| IBIS file stm32h523_533_lqfp144.ibs
[IBIS ver] 4.2
[File name] stm32h523_533_lqfp144.ibs
[File Rev] 0.2
[Date] 07-05-2024
[Source] Data Created at STMicroelectronics
[Notes]  File originated from ELDO simulations.
[Disclaimer]  This information is for modeling purpose only and is
   not guaranteed. The information is subject to change without
   notice.
[Copyright] Copyright 2024 STMicroelectronics Inc.
|   Component stm32h523_533_lqfp144
[Component] stm32h523_533_lqfp144
[Manufacturer] STMicroelectronics
[Package]
| variable   typ   min   max
R_pkg  0  NA  NA
L_pkg  0  NA  NA
C_pkg  0  NA  NA
[Pin]   signal_name   model_name
1  PE2  io8_ft_i3c_spi
2  PE3  io8_ft_i3c_spi
3  PE4  io8_ft_i3c_spi
4  PE5  io8_ft_i3c_spi
5  PE6  io8_ft_i3c_spi
6  VBAT  power
7  PC13  io8_ft_i3c_spi_v33
8  PC14-OSC32_IN  io_ft_tamp
9  PC15-OSC32_OUT  io_ft_tamp
10  PF0  io8_ft_i3c_spi
11  PF1  io8_ft_i3c_spi
12  PF2  io8_ft_i3c_spi
13  PF3  io8_ft_i3c_spi
14  PF4  io8_ft_i3c_spi
15  PF5  io8_ft_i3c_spi
16  VSS  gnd
17  VDD  power
18  PF6  io8_ft_i3c_spi
19  PF7  io8_ft_i3c_spi
20  PF8  io8_ft_i3c_spi
21  PF9  io8_ft_i3c_spi
22  PF10  io8_ft_i3c_spi
23  PH0-OSC_IN  io8_ft_i3c_spi
24  PH1-OSC_OUT  io8_ft_i3c_spi
25  NRST  ioreset_ft_v33
26  PC0  io8_ft_spi
27  PC1  io8_ft_spi
28  PC2  io8_ft_spi
29  PC3  io8_ft_spi
30  VDD  power
31  VSSA  nc
32  VREFP  nc
33  VDDA  nc
34  PA0  io8_ft_spi
35  PA1  io8_ft_spi_tamp
36  PA2  io8_ft_spi
37  PA3  io8_ft_spi
38  VSS  gnd
39  VDD  power
40  PA4  io8_ft_spi
41  PA5  io8_ft_spi
42  PA6  io8_ft_spi
43  PA7  io8_ft_spi
44  PC4  io8_ft_spi
45  PC5  io8_ft_spi
46  PB0  io8_ft_spi
47  PB1  io8_ft_spi
48  PB2  io8_ft_i3c_spi
49  PF11  io8_ft_spi
50  PF12  io8_ft_spi
51  VSS  gnd
52  VDD  power
53  PF13  io8_ft_spi
54  PF14  io8_ft_spi
55  PF15  io8_ft_i3c_spi
56  PG0  io8_ft_i3c_spi
57  PG1  io8_ft_i3c_spi
58  PE7  io8_ft_i3c_spi
59  PE8  io8_ft_i3c_spi
60  PE9  io8_ft_i3c_spi
61  VSS  gnd
62  VDD  power
63  PE10  io8_ft_i3c_spi
64  PE11  io8_ft_i3c_spi
65  PE12  io8_ft_i3c_spi
66  PE13  io8_ft_i3c_spi
67  PE14  io8_ft_i3c_spi
68  PE15  io8_ft_i3c_spi
69  PB10  io8_ft_i3c_spi
70  VCAP  nc
71  VSS  gnd
72  VDD  power
73  PB12  io8_ft_i3c_spi
74  PB13  nc
75  PB14  nc
76  PB15  io8_ft_spi
77  PD8  io8_ft_i3c_spi
78  PD9  io8_ft_i3c_spi
79  PD10  io8_ft_i3c_spi
80  PD11  io8_ft_i3c_spi
81  PD12  io8_ft_i3c_spi
82  PD13  io8_ft_i3c_spi
83  VSS  gnd
84  VDD  power
85  PD14  io8_ft_i3c_spi
86  PD15  io8_ft_i3c_spi
87  PG2  io8_ft_i3c_spi
88  PG3  io8_ft_i3c_spi
89  PG4  io8_ft_i3c_spi
90  PG5  io8_ft_i3c_spi
91  PG6  io8_ft_i3c_spi
92  PG7  io8_ft_i3c_spi
93  PG8  io8_ft_i3c_spi
94  VSS  gnd
95  VDD  power
96  PC6  io8_ft_i3c_spi
97  PC7  io8_ft_i3c_spi
98  PC8  io8_ft_i3c_spi
99  PC9  io8_ft_i3c_spi
100  PA8  io8_ft_i3c_spi
101  PA9  io8_ft_i3c_spi
102  PA10  io8_ft_i3c_spi
103  PA11  io8usb_ft_i3c_spi_phy
104  PA12  io8usb_ft_i3c_spi_phy
105  PA13  io8_ft_i3c_spi
106  VDDUSB  power
107  VSS  gnd
108  VDD  power
109  PA14  io8_ft_i3c_spi
110  PA15  io8_ft_i3c_spi
111  PC10  io8_ft_i3c_spi
112  PC11  io8_ft_i3c_spi
113  PC12  io8_ft_i3c_spi
114  PD0  io8_ft_i3c_spi
115  PD1  io8_ft_i3c_spi
116  PD2  io8_ft_i3c_spi
117  PD3  io8_ft_i3c_spi
118  PD4  io8_ft_i3c_spi
119  PD5  io8_ft_i3c_spi
120  VSS  gnd
121  VDDIO2  power
122  PD6  io8_ft_i3c_spi
123  PD7  io8_ft_i3c_spi
124  PG9  io8_ft_i3c_spi
125  PG10  io8_ft_i3c_spi
126  PG11  io8_ft_i3c_spi
127  PG12  io8_ft_i3c_spi
128  PG13  io8_ft_i3c_spi
129  PG14  io8_ft_i3c_spi
130  VSS  gnd
131  VDD  power
132  PG15  io8_ft_i3c_spi
133  PB3  io8_ft_i3c_spi
134  PB4  io8_ft_i3c_spi
135  PB5  io8_ft_i3c_spi
136  PB6  io8_ft_i3c_spi
137  PB7  io8_ft_i3c_spi
138  BOOT0  vpphv
139  PB8  io8_ft_i3c_spi
140  PB9  io8_ft_i3c_spi
141  PE0  io8_ft_i3c_spi
142  VCAP  nc
143  VSS  gnd
144  VDD  power
[Package Model]   478-lqfp-20x20-144-240315
[Pin Mapping]   pulldown_ref   pullup_ref   | Comment
1  gndio  vddio
2  gndio  vddio
3  gndio  vddio
4  gndio  vddio
5  gndio  vddio
6  nc  vsw
7  gndio  vddio  | Depending on IO usage
| 7  gndio  vsw  | Depending on IO usage
8  gndio  vddio  | Depending on IO usage
| 8  gndio  vsw  | Depending on IO usage
9  gndio  vddio  | Depending on IO usage
| 9  gndio  vsw  | Depending on IO usage
10  gndio  vddio
11  gndio  vddio
12  gndio  vddio
13  gndio  vddio
14  gndio  vddio
15  gndio  vddio
16  gndio  nc
17  nc  vddio
18  gndio  vddio
19  gndio  vddio
20  gndio  vddio
21  gndio  vddio
22  gndio  vddio
23  gndio  vddio
24  gndio  vddio
25  gndio  vddio
26  gndio  vddio
27  gndio  vddio
28  gndio  vddio
29  gndio  vddio
30  nc  vddio
31  nc  nc
32  nc  nc
33  nc  nc
34  gndio  vddio
35  gndio  vddio
36  gndio  vddio
37  gndio  vddio
38  gndio  nc
39  nc  vddio
40  gndio  vddio
41  gndio  vddio
42  gndio  vddio
43  gndio  vddio
44  gndio  vddio
45  gndio  vddio
46  gndio  vddio
47  gndio  vddio
48  gndio  vddio
49  gndio  vddio
50  gndio  vddio
51  gndio  nc
52  nc  vddio
53  gndio  vddio
54  gndio  vddio
55  gndio  vddio
56  gndio  vddio
57  gndio  vddio
58  gndio  vddio
59  gndio  vddio
60  gndio  vddio
61  gndio  nc
62  nc  vddio
63  gndio  vddio
64  gndio  vddio
65  gndio  vddio
66  gndio  vddio
67  gndio  vddio
68  gndio  vddio
69  gndio  vddio
70  nc  nc
71  gndio  nc
72  nc  vddio
73  gndio  vddio
74  nc  nc
75  nc  nc
76  gndio  vddio
77  gndio  vddio
78  gndio  vddio
79  gndio  vddio
80  gndio  vddio
81  gndio  vddio
82  gndio  vddio
83  gndio  nc
84  nc  vddio
85  gndio  vddio
86  gndio  vddio
87  gndio  vddio
88  gndio  vddio
89  gndio  vddio
90  gndio  vddio
91  gndio  vddio
92  gndio  vddio
93  gndio  vddio
94  gndio  nc
95  nc  vddio
96  gndio  vddio
97  gndio  vddio
98  gndio  vddio
99  gndio  vddio
100  gndio  vddio
101  gndio  vddio
102  gndio  vddio
103  gndio  vddusb  | Depending on IO usage
| 103  gndio  vddio  | Depending on IO usage
104  gndio  vddusb  | Depending on IO usage
| 104  gndio  vddio  | Depending on IO usage
105  gndio  vddio
106  nc  vddusb
107  gndio  nc
108  nc  vddio
109  gndio  vddio
110  gndio  vddio
111  gndio  vddio
112  gndio  vddio
113  gndio  vddio
114  gndio  vddio
115  gndio  vddio
116  gndio  vddio
117  gndio  vddio
118  gndio  vddio
119  gndio  vddio
120  gndio  nc
121  nc  vddmmc
122  gndio  vddmmc
123  gndio  vddmmc
124  gndio  vddmmc
125  gndio  vddmmc
126  gndio  vddmmc
127  gndio  vddmmc
128  gndio  vddmmc
129  gndio  vddmmc
130  gndio  nc
131  nc  vddio
132  gndio  vddio
133  gndio  vddio
134  gndio  vddio
135  gndio  vddio
136  gndio  vddio
137  gndio  vddio
138  gndio  vddio
139  gndio  vddmmc
140  gndio  vddmmc
141  gndio  vddio
142  nc  nc
143  gndio  nc
144  nc  vddio
|[Diff Pin]  inv_pin  vdiff  tdelay_typ  tdelay_min  tdelay_max
|104  103  NA  NA  NA  NA
[Model Selector] io8_ft_i3c_spi
io8_ft_spi_ls_1v2 "GPIO SPI - 5V tolerant - low speed - 1.2V range"
io8_ft_spi_ls_1v8 "GPIO SPI - 5V tolerant - low speed - 1.8V range"
io8_ft_spi_ls_3v3 "GPIO SPI - 5V tolerant - low speed - 3.3V range"
io8_ft_spi_ms_1v2 "GPIO SPI - 5V tolerant - med speed - 1.2V range"
io8_ft_spi_ms_1v8 "GPIO SPI - 5V tolerant - med speed - 1.8V range"
io8_ft_spi_ms_3v3 "GPIO SPI - 5V tolerant - med speed - 3.3V range"
io8_ft_spi_fs_1v2 "GPIO SPI - 5V tolerant - fast speed - 1.2V range"
io8_ft_spi_fs_1v8 "GPIO SPI - 5V tolerant - fast speed - 1.8V range"
io8_ft_spi_fs_3v3 "GPIO SPI - 5V tolerant - fast speed - 3.3V range"
io8_ft_spi_hs_1v2 "GPIO SPI - 5V tolerant - high speed - 1.2V range"
io8_ft_spi_hs_1v8 "GPIO SPI - 5V tolerant - high speed - 1.8V range"
io8_ft_spi_hs_3v3 "GPIO SPI - 5V tolerant - high speed - 3.3V range"
io8_ft_hslv_spi_ls_1v2 "GPIO SPI low volt opt - 5V tolerant - low speed - 1.2V range"
io8_ft_hslv_spi_ls_1v8 "GPIO SPI low volt opt - 5V tolerant - low speed - 1.8V range"
io8_ft_hslv_spi_ls_2v5 "GPIO SPI low volt opt - 5V tolerant - low speed - 2.5V range"
io8_ft_hslv_spi_ms_1v2 "GPIO SPI low volt opt - 5V tolerant - med speed - 1.2V range"
io8_ft_hslv_spi_ms_1v8 "GPIO SPI low volt opt - 5V tolerant - med speed - 1.8V range"
io8_ft_hslv_spi_ms_2v5 "GPIO SPI low volt opt - 5V tolerant - med speed - 2.5V range"
io8_ft_hslv_spi_fs_1v2 "GPIO SPI low volt opt - 5V tolerant - fast speed - 1.2V range"
io8_ft_hslv_spi_fs_1v8 "GPIO SPI low volt opt - 5V tolerant - fast speed - 1.8V range"
io8_ft_hslv_spi_fs_2v5 "GPIO SPI low volt opt - 5V tolerant - fast speed - 2.5V range"
io8_ft_hslv_spi_hs_1v2 "GPIO SPI low volt opt - 5V tolerant - high speed - 1.2V range"
io8_ft_hslv_spi_hs_1v8 "GPIO SPI low volt opt - 5V tolerant - high speed - 1.8V range"
io8_ft_hslv_spi_hs_2v5 "GPIO SPI low volt opt - 5V tolerant - high speed - 2.5V range"
io8_ft_i3c_spi_ls_1v2 "GPIO SPI with I3C open-drain - 5V tolerant - low speed - 1.2V range"
io8_ft_i3c_spi_ls_1v8 "GPIO SPI with I3C open-drain - 5V tolerant - low speed - 1.8V range"
io8_ft_i3c_spi_ls_3v3 "GPIO SPI with I3C open-drain - 5V tolerant - low speed - 3.3V range"
io8_ft_i3c_spi_ms_1v2 "GPIO SPI with I3C open-drain - 5V tolerant - med speed - 1.2V range"
io8_ft_i3c_spi_ms_1v8 "GPIO SPI with I3C open-drain - 5V tolerant - med speed - 1.8V range"
io8_ft_i3c_spi_ms_3v3 "GPIO SPI with I3C open-drain - 5V tolerant - med speed - 3.3V range"
io8_ft_i3c_spi_fs_1v2 "GPIO SPI with I3C open-drain - 5V tolerant - fast speed - 1.2V range"
io8_ft_i3c_spi_fs_1v8 "GPIO SPI with I3C open-drain - 5V tolerant - fast speed - 1.8V range"
io8_ft_i3c_spi_fs_3v3 "GPIO SPI with I3C open-drain - 5V tolerant - fast speed - 3.3V range"
io8_ft_i3c_spi_hs_1v2 "GPIO SPI with I3C open-drain - 5V tolerant - high speed - 1.2V range"
io8_ft_i3c_spi_hs_1v8 "GPIO SPI with I3C open-drain - 5V tolerant - high speed - 1.8V range"
io8_ft_i3c_spi_hs_3v3 "GPIO SPI with I3C open-drain - 5V tolerant - high speed - 3.3V range"
io8_ft_hslv_i3c_spi_ls_1v2 "GPIO SPI low volt opt with I3C open-drain - 5V tolerant - low speed - 1.2V range"
io8_ft_hslv_i3c_spi_ls_1v8 "GPIO SPI low volt opt with I3C open-drain - 5V tolerant - low speed - 1.8V range"
io8_ft_hslv_i3c_spi_ls_2v5 "GPIO SPI low volt opt with I3C open-drain - 5V tolerant - low speed - 2.5V range"
io8_ft_hslv_i3c_spi_ms_1v2 "GPIO SPI low volt opt with I3C open-drain - 5V tolerant - med speed - 1.2V range"
io8_ft_hslv_i3c_spi_ms_1v8 "GPIO SPI low volt opt with I3C open-drain - 5V tolerant - med speed - 1.8V range"
io8_ft_hslv_i3c_spi_ms_2v5 "GPIO SPI low volt opt with I3C open-drain - 5V tolerant - med speed - 2.5V range"
io8_ft_hslv_i3c_spi_fs_1v2 "GPIO SPI low volt opt with I3C open-drain - 5V tolerant - fast speed - 1.2V range"
io8_ft_hslv_i3c_spi_fs_1v8 "GPIO SPI low volt opt with I3C open-drain - 5V tolerant - fast speed - 1.8V range"
io8_ft_hslv_i3c_spi_fs_2v5 "GPIO SPI low volt opt with I3C open-drain - 5V tolerant - fast speed - 2.5V range"
io8_ft_hslv_i3c_spi_hs_1v2 "GPIO SPI low volt opt with I3C open-drain - 5V tolerant - high speed - 1.2V range"
io8_ft_hslv_i3c_spi_hs_1v8 "GPIO SPI low volt opt with I3C open-drain - 5V tolerant - high speed - 1.8V range"
io8_ft_hslv_i3c_spi_hs_2v5 "GPIO SPI low volt opt with I3C open-drain - 5V tolerant - high speed - 2.5V range"
io8_ft_i3c_fmp_spi_3v3 "GPIO SPI with I3C fm+ open-drain - 5V tolerant - 3.3V range"
io8_ft_i3c_fmp_spi_1v8 "GPIO SPI with I3C fm+ open-drain - 5V tolerant - 1.8V range"
io8_ft_i3c_fmp_spi_1v2 "GPIO SPI with I3C fm+ open-drain - 5V tolerant - 1.2V range"
[Model Selector] io8_ft_i3c_spi_v33
io8_ft_spi_v33_ls_1v2 ""GPIO SPI V33 - 5V tolerant - low speed - 1.2V range"
io8_ft_spi_v33_ls_1v8 ""GPIO SPI V33 - 5V tolerant - low speed - 1.8V range"
io8_ft_spi_v33_ls_3v3 ""GPIO SPI V33 - 5V tolerant - low speed - 3.3V range"
io8_ft_spi_v33_ms_1v2 ""GPIO SPI V33 - 5V tolerant - med speed - 1.2V range"
io8_ft_spi_v33_ms_1v8 ""GPIO SPI V33 - 5V tolerant - med speed - 1.8V range"
io8_ft_spi_v33_ms_3v3 ""GPIO SPI V33 - 5V tolerant - med speed - 3.3V range"
io8_ft_spi_v33_fs_1v2 ""GPIO SPI V33 - 5V tolerant - fast speed - 1.2V range
io8_ft_spi_v33_fs_1v8 ""GPIO SPI V33 - 5V tolerant - fast speed - 1.8V range
io8_ft_spi_v33_fs_3v3 ""GPIO SPI V33 - 5V tolerant - fast speed - 3.3V range
io8_ft_spi_v33_hs_1v2 ""GPIO SPI V33 - 5V tolerant - high speed - 1.2V range
io8_ft_spi_v33_hs_1v8 ""GPIO SPI V33 - 5V tolerant - high speed - 1.8V range
io8_ft_spi_v33_hs_3v3 ""GPIO SPI V33 - 5V tolerant - high speed - 3.3V range
io8_ft_hslv_spi_v33_ls_1v2 "GPIO SPI V33 low volt opt - 5V tolerant - low speed - 1.2V range""
io8_ft_hslv_spi_v33_ls_1v8 "GPIO SPI V33 low volt opt - 5V tolerant - low speed - 1.8V range""
io8_ft_hslv_spi_v33_ls_2v5 "GPIO SPI V33 low volt opt - 5V tolerant - low speed - 2.5V range""
io8_ft_hslv_spi_v33_ms_1v2 "GPIO SPI V33 low volt opt - 5V tolerant - med speed - 1.2V range""
io8_ft_hslv_spi_v33_ms_1v8 "GPIO SPI V33 low volt opt - 5V tolerant - med speed - 1.8V range""
io8_ft_hslv_spi_v33_ms_2v5 "GPIO SPI V33 low volt opt - 5V tolerant - med speed - 2.5V range""
io8_ft_hslv_spi_v33_fs_1v2 "GPIO SPI V33 low volt opt - 5V tolerant - fast speed - 1.2V range"
io8_ft_hslv_spi_v33_fs_1v8 "GPIO SPI V33 low volt opt - 5V tolerant - fast speed - 1.8V range"
io8_ft_hslv_spi_v33_fs_2v5 "GPIO SPI V33 low volt opt - 5V tolerant - fast speed - 2.5V range"
io8_ft_hslv_spi_v33_hs_1v2 "GPIO SPI V33 low volt opt - 5V tolerant - high speed - 1.2V range"
io8_ft_hslv_spi_v33_hs_1v8 "GPIO SPI V33 low volt opt - 5V tolerant - high speed - 1.8V range"
io8_ft_hslv_spi_v33_hs_2v5 "GPIO SPI V33 low volt opt - 5V tolerant - high speed - 2.5V range"
io8_ft_i3c_spi_v33_ls_1v2 "GPIO SPI V33 with I3C open-drain - 5V tolerant - low speed - 1.2V range"
io8_ft_i3c_spi_v33_ls_1v8 "GPIO SPI V33 with I3C open-drain - 5V tolerant - low speed - 1.8V range"
io8_ft_i3c_spi_v33_ls_3v3 "GPIO SPI V33 with I3C open-drain - 5V tolerant - low speed - 3.3V range"
io8_ft_i3c_spi_v33_ms_1v2 "GPIO SPI V33 with I3C open-drain - 5V tolerant - med speed - 1.2V range"
io8_ft_i3c_spi_v33_ms_1v8 "GPIO SPI V33 with I3C open-drain - 5V tolerant - med speed - 1.8V range"
io8_ft_i3c_spi_v33_ms_3v3 "GPIO SPI V33 with I3C open-drain - 5V tolerant - med speed - 3.3V range"
io8_ft_i3c_spi_v33_fs_1v2 "GPIO SPI V33 with I3C open-drain - 5V tolerant - fast speed - 1.2V range"
io8_ft_i3c_spi_v33_fs_1v8 "GPIO SPI V33 with I3C open-drain - 5V tolerant - fast speed - 1.8V range"
io8_ft_i3c_spi_v33_fs_3v3 "GPIO SPI V33 with I3C open-drain - 5V tolerant - fast speed - 3.3V range"
io8_ft_i3c_spi_v33_hs_1v2 "GPIO SPI V33 with I3C open-drain - 5V tolerant - high speed - 1.2V range"
io8_ft_i3c_spi_v33_hs_1v8 "GPIO SPI V33 with I3C open-drain - 5V tolerant - high speed - 1.8V range"
io8_ft_i3c_spi_v33_hs_3v3 "GPIO SPI V33 with I3C open-drain - 5V tolerant - high speed - 3.3V range"
io8_ft_hslv_i3c_spi_v33_ls_1v2 "GPIO SPI V33 low volt opt with I3C open-drain - 5V tolerant - low speed - 1.2V range"
io8_ft_hslv_i3c_spi_v33_ls_1v8 "GPIO SPI V33 low volt opt with I3C open-drain - 5V tolerant - low speed - 1.8V range"
io8_ft_hslv_i3c_spi_v33_ls_2v5 "GPIO SPI V33 low volt opt with I3C open-drain - 5V tolerant - low speed - 2.5V range"
io8_ft_hslv_i3c_spi_v33_ms_1v2 "GPIO SPI V33 low volt opt with I3C open-drain - 5V tolerant - med speed - 1.2V range"
io8_ft_hslv_i3c_spi_v33_ms_1v8 "GPIO SPI V33 low volt opt with I3C open-drain - 5V tolerant - med speed - 1.8V range"
io8_ft_hslv_i3c_spi_v33_ms_2v5 "GPIO SPI V33 low volt opt with I3C open-drain - 5V tolerant - med speed - 2.5V range"
io8_ft_hslv_i3c_spi_v33_fs_1v2 "GPIO SPI V33 low volt opt with I3C open-drain - 5V tolerant - fast speed - 1.2V range"
io8_ft_hslv_i3c_spi_v33_fs_1v8 "GPIO SPI V33 low volt opt with I3C open-drain - 5V tolerant - fast speed - 1.8V range"
io8_ft_hslv_i3c_spi_v33_fs_2v5 "GPIO SPI V33 low volt opt with I3C open-drain - 5V tolerant - fast speed - 2.5V range"
io8_ft_hslv_i3c_spi_v33_hs_1v2 "GPIO SPI V33 low volt opt with I3C open-drain - 5V tolerant - high speed - 1.2V range"
io8_ft_hslv_i3c_spi_v33_hs_1v8 "GPIO SPI V33 low volt opt with I3C open-drain - 5V tolerant - high speed - 1.8V range"
io8_ft_hslv_i3c_spi_v33_hs_2v5 "GPIO SPI V33 low volt opt with I3C open-drain - 5V tolerant - high speed - 2.5V range"
io8_ft_i3c_fmp_spi_v33_3v3 "GPIO SPI V33 with I3C fm+ open-drain - 5V tolerant - 3.3V range"
io8_ft_i3c_fmp_spi_v33_1v8 "GPIO SPI V33 with I3C fm+ open-drain - 5V tolerant - 1.8V range"
io8_ft_i3c_fmp_spi_v33_1v2 "GPIO SPI V33 with I3C fm+ open-drain - 5V tolerant - 1.2V range"
[Model Selector] io8_ft_spi
io8_ft_spi_ls_1v2 "GPIO SPI - 5V tolerant - low speed - 1.2V range"
io8_ft_spi_ls_1v8 "GPIO SPI - 5V tolerant - low speed - 1.8V range"
io8_ft_spi_ls_3v3 "GPIO SPI - 5V tolerant - low speed - 3.3V range"
io8_ft_spi_ms_1v2 "GPIO SPI- 5V tolerant - med speed - 1.2V range"
io8_ft_spi_ms_1v8 "GPIO SPI- 5V tolerant - med speed - 1.8V range"
io8_ft_spi_ms_3v3 "GPIO SPI- 5V tolerant - med speed - 3.3V range"
io8_ft_spi_fs_1v2 "GPIO SPI- 5V tolerant - fast speed - 1.2V range"
io8_ft_spi_fs_1v8 "GPIO SPI- 5V tolerant - fast speed - 1.8V range"
io8_ft_spi_fs_3v3 "GPIO SPI- 5V tolerant - fast speed - 3.3V range"
io8_ft_spi_hs_1v2 "GPIO SPI- 5V tolerant - high speed - 1.2V range"
io8_ft_spi_hs_1v8 "GPIO SPI- 5V tolerant - high speed - 1.8V range"
io8_ft_spi_hs_3v3 "GPIO SPI- 5V tolerant - high speed - 3.3V range"
io8_ft_hslv_spi_ls_1v2 "GPIO SPI low volt opt - 5V tolerant - low speed - 1.2V range"
io8_ft_hslv_spi_ls_1v8 "GPIO SPI low volt opt - 5V tolerant - low speed - 1.8V range"
io8_ft_hslv_spi_ls_2v5 "GPIO SPI low volt opt - 5V tolerant - low speed - 2.5V range"
io8_ft_hslv_spi_ms_1v2 "GPIO SPI low volt opt - 5V tolerant - med speed - 1.2V range"
io8_ft_hslv_spi_ms_1v8 "GPIO SPI low volt opt - 5V tolerant - med speed - 1.8V range"
io8_ft_hslv_spi_ms_2v5 "GPIO SPI low volt opt - 5V tolerant - med speed - 2.5V range"
io8_ft_hslv_spi_fs_1v2 "GPIO SPI low volt opt - 5V tolerant - fast speed - 1.2V range"
io8_ft_hslv_spi_fs_1v8 "GPIO SPI low volt opt - 5V tolerant - fast speed - 1.8V range"
io8_ft_hslv_spi_fs_2v5 "GPIO SPI low volt opt - 5V tolerant - fast speed - 2.5V range"
io8_ft_hslv_spi_hs_1v2 "GPIO SPI low volt opt - 5V tolerant - high speed - 1.2V range"
io8_ft_hslv_spi_hs_1v8 "GPIO SPI low volt opt - 5V tolerant - high speed - 1.8V range"
io8_ft_hslv_spi_hs_2v5 "GPIO SPI low volt opt - 5V tolerant - high speed - 2.5V range"
[Model Selector] io8_ft_spi_tamp
io8_ft_spi_ls_1v2 "GPIO SPI - 5V tolerant - low speed - 1.2V range"
io8_ft_spi_ls_1v8 "GPIO SPI - 5V tolerant - low speed - 1.8V range"
io8_ft_spi_ls_3v3 "GPIO SPI- 5V tolerant - low speed - 3.3V range"
io8_ft_spi_ms_1v2 "GPIO SPI - 5V tolerant - med speed - 1.2V range"
io8_ft_spi_ms_1v8 "GPIO SPI - 5V tolerant - med speed - 1.8V range"
io8_ft_spi_ms_3v3 "GPIO SPI - 5V tolerant - med speed - 3.3V range"
io8_ft_spi_fs_1v2 "GPIO SPI - 5V tolerant - fast speed - 1.2V range"
io8_ft_spi_fs_1v8 "GPIO SPI - 5V tolerant - fast speed - 1.8V range"
io8_ft_spi_fs_3v3 "GPIO SPI - 5V tolerant - fast speed - 3.3V range"
io8_ft_spi_hs_1v2 "GPIO SPI - 5V tolerant - high speed - 1.2V range"
io8_ft_spi_hs_1v8 "GPIO SPI - 5V tolerant - high speed - 1.8V range"
io8_ft_spi_hs_3v3 "GPIO SPI - 5V tolerant - high speed - 3.3V range"
io8_ft_hslv_spi_ls_1v2 "GPIO SPI low volt opt - 5V tolerant - low speed - 1.2V range"
io8_ft_hslv_spi_ls_1v8 "GPIO SPI low volt opt - 5V tolerant - low speed - 1.8V range"
io8_ft_hslv_spi_ls_2v5 "GPIO SPI low volt opt - 5V tolerant - low speed - 2.5V range"
io8_ft_hslv_spi_ms_1v2 "GPIO SPI low volt opt - 5V tolerant - med speed - 1.2V range"
io8_ft_hslv_spi_ms_1v8 "GPIO SPI low volt opt - 5V tolerant - med speed - 1.8V range"
io8_ft_hslv_spi_ms_2v5 "GPIO SPI low volt opt - 5V tolerant - med speed - 2.5V range"
io8_ft_hslv_spi_fs_1v2 "GPIO SPI low volt opt - 5V tolerant - fast speed - 1.2V range"
io8_ft_hslv_spi_fs_1v8 "GPIO SPI low volt opt - 5V tolerant - fast speed - 1.8V range"
io8_ft_hslv_spi_fs_2v5 "GPIO SPI low volt opt - 5V tolerant - fast speed - 2.5V range"
io8_ft_hslv_spi_hs_1v2 "GPIO SPI low volt opt - 5V tolerant - high speed - 1.2V range"
io8_ft_hslv_spi_hs_1v8 "GPIO SPI low volt opt - 5V tolerant - high speed - 1.8V range"
io8_ft_hslv_spi_hs_2v5 "GPIO SPI low volt opt - 5V tolerant - high speed - 2.5V range
io8_ft_tamp_v33_1v2 "IO tamper - 5V tolerant - 1.2V range"
io8_ft_tamp_v33_1v8 "IO tamper - 5V tolerant - 1.8V range"
io8_ft_tamp_v33_3v3 "IO tamper - 5V tolerant - 3.3V range"
[Model Selector] io8usb_ft_i3c_spi_phy
io8_ft_spi_ls_1v2 "GPIO SPI - 5V tolerant - low speed - 1.2V range"
io8_ft_spi_ls_1v8 "GPIO SPI - 5V tolerant - low speed - 1.8V range"
io8_ft_spi_ls_3v3 "GPIO SPI - 5V tolerant - low speed - 3.3V range"
io8_ft_spi_ms_1v2 "GPIO SPI - 5V tolerant - med speed - 1.2V range"
io8_ft_spi_ms_1v8 "GPIO SPI - 5V tolerant - med speed - 1.8V range"
io8_ft_spi_ms_3v3 "GPIO SPI - 5V tolerant - med speed - 3.3V range"
io8_ft_spi_fs_1v2 "GPIO SPI - 5V tolerant - fast speed - 1.2V range"
io8_ft_spi_fs_1v8 "GPIO SPI - 5V tolerant - fast speed - 1.8V range"
io8_ft_spi_fs_3v3 "GPIO SPI - 5V tolerant - fast speed - 3.3V range"
io8_ft_spi_hs_1v2 "GPIO SPI - 5V tolerant - high speed - 1.2V range"
io8_ft_spi_hs_1v8 "GPIO SPI - 5V tolerant - high speed - 1.8V range"
io8_ft_spi_hs_3v3 "GPIO SPI - 5V tolerant - high speed - 3.3V range"
io8_ft_hslv_spi_ls_1v2 "GPIO SPI low volt opt - 5V tolerant - low speed - 1.2V range"
io8_ft_hslv_spi_ls_1v8 "GPIO SPI low volt opt - 5V tolerant - low speed - 1.8V range"
io8_ft_hslv_spi_ls_2v5 "GPIO SPI low volt opt - 5V tolerant - low speed - 2.5V range"
io8_ft_hslv_spi_ms_1v2 "GPIO SPI low volt opt - 5V tolerant - med speed - 1.2V range"
io8_ft_hslv_spi_ms_1v8 "GPIO SPI low volt opt - 5V tolerant - med speed - 1.8V range"
io8_ft_hslv_spi_ms_2v5 "GPIO SPI low volt opt - 5V tolerant - med speed - 2.5V range"
io8_ft_hslv_spi_fs_1v2 "GPIO SPI low volt opt - 5V tolerant - fast speed - 1.2V range"
io8_ft_hslv_spi_fs_1v8 "GPIO SPI low volt opt - 5V tolerant - fast speed - 1.8V range"
io8_ft_hslv_spi_fs_2v5 "GPIO SPI low volt opt - 5V tolerant - fast speed - 2.5V range"
io8_ft_hslv_spi_hs_1v2 "GPIO SPI low volt opt - 5V tolerant - high speed - 1.2V range"
io8_ft_hslv_spi_hs_1v8 "GPIO SPI low volt opt - 5V tolerant - high speed - 1.8V range"
io8_ft_hslv_spi_hs_2v5 "GPIO SPI low volt opt - 5V tolerant - high speed - 2.5V range"
io8_ft_i3c_spi_ls_1v2 "GPIO SPI  with I3C open-drain - 5V tolerant - low speed - 1.2V range"
io8_ft_i3c_spi_ls_1v8 "GPIO SPI  with I3C open-drain - 5V tolerant - low speed - 1.8V range"
io8_ft_i3c_spi_ls_3v3 "GPIO SPI  with I3C open-drain - 5V tolerant - low speed - 3.3V range"
io8_ft_i3c_spi_ms_1v2 "GPIO SPI  with I3C open-drain - 5V tolerant - med speed - 1.2V range"
io8_ft_i3c_spi_ms_1v8 "GPIO SPI  with I3C open-drain - 5V tolerant - med speed - 1.8V range"
io8_ft_i3c_spi_ms_3v3 "GPIO SPI  with I3C open-drain - 5V tolerant - med speed - 3.3V range"
io8_ft_i3c_spi_fs_1v2 "GPIO SPI  with I3C open-drain - 5V tolerant - fast speed - 1.2V range"
io8_ft_i3c_spi_fs_1v8 "GPIO SPI  with I3C open-drain - 5V tolerant - fast speed - 1.8V range"
io8_ft_i3c_spi_fs_3v3 "GPIO SPI  with I3C open-drain - 5V tolerant - fast speed - 3.3V range"
io8_ft_i3c_spi_hs_1v2 "GPIO SPI  with I3C open-drain - 5V tolerant - high speed - 1.2V range"
io8_ft_i3c_spi_hs_1v8 "GPIO SPI  with I3C open-drain - 5V tolerant - high speed - 1.8V range"
io8_ft_i3c_spi_hs_3v3 "GPIO SPI  with I3C open-drain - 5V tolerant - high speed - 3.3V range"
io8_ft_hslv_i3c_spi_ls_1v2 "GPIO SPI  low volt opt with I3C open-drain - 5V tolerant - low speed - 1.2V range"
io8_ft_hslv_i3c_spi_ls_1v8 "GPIO SPI  low volt opt with I3C open-drain - 5V tolerant - low speed - 1.8V range"
io8_ft_hslv_i3c_spi_ls_2v5 "GPIO SPI  low volt opt with I3C open-drain - 5V tolerant - low speed - 2.5V range"
io8_ft_hslv_i3c_spi_ms_1v2 "GPIO SPI  low volt opt with I3C open-drain - 5V tolerant - med speed - 1.2V range"
io8_ft_hslv_i3c_spi_ms_1v8 "GPIO SPI  low volt opt with I3C open-drain - 5V tolerant - med speed - 1.8V range"
io8_ft_hslv_i3c_spi_ms_2v5 "GPIO SPI  low volt opt with I3C open-drain - 5V tolerant - med speed - 2.5V range"
io8_ft_hslv_i3c_spi_fs_1v2 "GPIO SPI  low volt opt with I3C open-drain - 5V tolerant - fast speed - 1.2V range"
io8_ft_hslv_i3c_spi_fs_1v8 "GPIO SPI  low volt opt with I3C open-drain - 5V tolerant - fast speed - 1.8V range"
io8_ft_hslv_i3c_spi_fs_2v5 "GPIO SPI  low volt opt with I3C open-drain - 5V tolerant - fast speed - 2.5V range"
io8_ft_hslv_i3c_spi_hs_1v2 "GPIO SPI  low volt opt with I3C open-drain - 5V tolerant - high speed - 1.2V range"
io8_ft_hslv_i3c_spi_hs_1v8 "GPIO SPI  low volt opt with I3C open-drain - 5V tolerant - high speed - 1.8V range"
io8_ft_hslv_i3c_spi_hs_2v5 "GPIO SPI  low volt opt with I3C open-drain - 5V tolerant - high speed - 2.5V range"
io8_ft_i3c_fmp_spi_3v3 "GPIO SPI  with I3C fm+ open-drain - 5V tolerant - 3.3V range"
io8_ft_i3c_fmp_spi_1v8 "GPIO SPI  with I3C fm+ open-drain - 5V tolerant - 1.8V range"
io8_ft_i3c_fmp_spi_1v2 "GPIO SPI  with I3C fm+ open-drain - 5V tolerant - 1.2V range"
io8usb_ft_phy_ls_2v5 "USB PHY - 5V tolerant - low speed - 2.5V range"
io8usb_ft_phy_ls_3v3 "USB PHY - 5V tolerant - low speed - 3.3V range
io8usb_ft_phy_fs_2v5 "USB PHY - 5V tolerant - fast speed - 2.5V range"
io8usb_ft_phy_fs_3v3 "USB PHY - 5V tolerant - fast speed - 3.3V range"
[Model Selector] io_ft_tamp
io_ft_tamp_3v3 "IO tamper - 5V tolerant - 3.3V range"
io_ft_tamp_1v8 "IO tamper - 5V tolerant - 1.8V range"
io_ft_tamp_1v2 "IO tamper - 5V tolerant - 1.2V range"
[Model Selector] ioreset_ft_v33
ioreset_ft_v33_1v2 "Reset PAD. 5V tolerant. 1.2V range"
ioreset_ft_v33_1v8 "Reset PAD. 5V tolerant. 1.8V range"
ioreset_ft_v33_3v3 "Reset PAD. 5V tolerant. 3.3V range"
[Model Selector] vpphv
vpphv_1v2 "Flash Test cell v33 = 1.2 V range"
vpphv_1v8 "Flash Test cell v33 = 1.8 V range"
vpphv_3v3 "Flash Test cell v33 = 3.3 V range"
[Define Package Model]  478-lqfp-20x20-144-240315
[Manufacturer]  Unknown
[OEM]  Unknown
[Description]  None
[Number Of Pins]  137
[Pin Numbers]
| Pin Num   Terminal Name
25 | NRST
34 | PA0
35 | PA1
36 | PA2
37 | PA3
40 | PA4
41 | PA5
42 | PA6
43 | PA7
100 | PA8
101 | PA9
102 | PA10
103 | PA11
104 | PA12
105 | PA13
109 | PA14
110 | PA15
46 | PB0
47 | PB1
48 | PB2
133 | PB3
134 | PB4
135 | PB5
136 | PB6
137 | PB7
139 | PB8
140 | PB9
69 | PB10
73 | PB12
74 | PB13
75 | PB14
76 | PB15
26 | PC0
27 | PC1
28 | PC2
29 | PC3
44 | PC4
45 | PC5
96 | PC6
97 | PC7
98 | PC8
99 | PC9
111 | PC10
112 | PC11
113 | PC12
7 | PC13
8 | PC14-OSC32_IN
9 | PC15-OSC32_OUT
114 | PD0
115 | PD1
116 | PD2
117 | PD3
118 | PD4
119 | PD5
122 | PD6
123 | PD7
77 | PD8
78 | PD9
79 | PD10
80 | PD11
81 | PD12
82 | PD13
85 | PD14
86 | PD15
141 | PE0
1 | PE2
2 | PE3
3 | PE4
4 | PE5
5 | PE6
58 | PE7
59 | PE8
60 | PE9
63 | PE10
64 | PE11
65 | PE12
66 | PE13
67 | PE14
68 | PE15
10 | PF0
11 | PF1
12 | PF2
13 | PF3
14 | PF4
15 | PF5
18 | PF6
19 | PF7
20 | PF8
21 | PF9
22 | PF10
49 | PF11
50 | PF12
53 | PF13
54 | PF14
55 | PF15
56 | PG0
57 | PG1
87 | PG2
88 | PG3
89 | PG4
90 | PG5
91 | PG6
92 | PG7
93 | PG8
124 | PG9
125 | PG10
126 | PG11
127 | PG12
128 | PG13
129 | PG14
132 | PG15
23 | PH0-OSC_IN
24 | PH1-OSC_OUT
6 | VBAT
70 | VCAP
142 | VCAP
72 | VDD
108 | VDD
17 | VDD
30 | VDD
39 | VDD
52 | VDD
62 | VDD
144 | VDD
84 | VDD
131 | VDD
95 | VDD
121 | VDDIO2
106 | VDDUSB
33 | VDDA
138 | BOOT0
32 | VREFP
51 | VSS
130 | VSS
94 | VSS
16 | VSS
31 | VSSA
|[Merged Pins]  16
|38  |  VSS
|61  |  VSS
|71  |  VSS
|83  |  VSS
|107  |  VSS
|120  |  VSS
|143  |  VSS
[Model Data]
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[End Model Data]
[End Package Model]
|End [Component]
| Models and submodels in the file (118): io8_ft_hslv_i3c_spi_fs_1v2 (I/O_open_drain), io8_ft_hslv_i3c_spi_fs_1v8 (I/O_open_drain), io8_ft_hslv_i3c_spi_fs_2v5 (I/O_open_drain), io8_ft_hslv_i3c_spi_hs_1v2 (I/O_open_drain), io8_ft_hslv_i3c_spi_hs_1v8 (I/O_open_drain), io8_ft_hslv_i3c_spi_hs_2v5 (I/O_open_drain), io8_ft_hslv_i3c_spi_ls_1v2 (I/O_open_drain), io8_ft_hslv_i3c_spi_ls_1v8 (I/O_open_drain), io8_ft_hslv_i3c_spi_ls_2v5 (I/O_open_drain), io8_ft_hslv_i3c_spi_ms_1v2 (I/O_open_drain), io8_ft_hslv_i3c_spi_ms_1v8 (I/O_open_drain), io8_ft_hslv_i3c_spi_ms_2v5 (I/O_open_drain), io8_ft_hslv_i3c_spi_v33_fs_1v2 (I/O_open_drain), io8_ft_hslv_i3c_spi_v33_fs_1v8 (I/O_open_drain), io8_ft_hslv_i3c_spi_v33_fs_2v5 (I/O_open_drain), io8_ft_hslv_i3c_spi_v33_hs_1v2 (I/O_open_drain), io8_ft_hslv_i3c_spi_v33_hs_1v8 (I/O_open_drain), io8_ft_hslv_i3c_spi_v33_hs_2v5 (I/O_open_drain), io8_ft_hslv_i3c_spi_v33_ls_1v2 (I/O_open_drain), io8_ft_hslv_i3c_spi_v33_ls_1v8 (I/O_open_drain), io8_ft_hslv_i3c_spi_v33_ls_2v5 (I/O_open_drain), io8_ft_hslv_i3c_spi_v33_ms_1v2 (I/O_open_drain), io8_ft_hslv_i3c_spi_v33_ms_1v8 (I/O_open_drain), io8_ft_hslv_i3c_spi_v33_ms_2v5 (I/O_open_drain), io8_ft_hslv_spi_fs_1v2 (I/O), io8_ft_hslv_spi_fs_1v8 (I/O), io8_ft_hslv_spi_fs_2v5 (I/O), io8_ft_hslv_spi_hs_1v2 (I/O), io8_ft_hslv_spi_hs_1v8 (I/O), io8_ft_hslv_spi_hs_2v5 (I/O), io8_ft_hslv_spi_ls_1v2 (I/O), io8_ft_hslv_spi_ls_1v8 (I/O), io8_ft_hslv_spi_ls_2v5 (I/O), io8_ft_hslv_spi_ms_1v2 (I/O), io8_ft_hslv_spi_ms_1v8 (I/O), io8_ft_hslv_spi_ms_2v5 (I/O), io8_ft_hslv_spi_v33_fs_1v2 (I/O), io8_ft_hslv_spi_v33_fs_1v8 (I/O), io8_ft_hslv_spi_v33_fs_2v5 (I/O), io8_ft_hslv_spi_v33_hs_1v2 (I/O), io8_ft_hslv_spi_v33_hs_1v8 (I/O), io8_ft_hslv_spi_v33_hs_2v5 (I/O), io8_ft_hslv_spi_v33_ls_1v2 (I/O), io8_ft_hslv_spi_v33_ls_1v8 (I/O), io8_ft_hslv_spi_v33_ls_2v5 (I/O), io8_ft_hslv_spi_v33_ms_1v2 (I/O), io8_ft_hslv_spi_v33_ms_1v8 (I/O), io8_ft_hslv_spi_v33_ms_2v5 (I/O), io8_ft_i3c_fmp_spi_1v2 (I/O_open_drain), io8_ft_i3c_fmp_spi_1v8 (I/O_open_drain), io8_ft_i3c_fmp_spi_3v3 (I/O_open_drain), io8_ft_i3c_fmp_spi_v33_1v2 (I/O_open_drain), io8_ft_i3c_fmp_spi_v33_1v8 (I/O_open_drain), io8_ft_i3c_fmp_spi_v33_3v3 (I/O_open_drain), io8_ft_i3c_spi_fs_1v2 (I/O_open_drain), io8_ft_i3c_spi_fs_1v8 (I/O_open_drain), io8_ft_i3c_spi_fs_3v3 (I/O_open_drain), io8_ft_i3c_spi_hs_1v2 (I/O_open_drain), io8_ft_i3c_spi_hs_1v8 (I/O_open_drain), io8_ft_i3c_spi_hs_3v3 (I/O_open_drain), io8_ft_i3c_spi_ls_1v2 (I/O_open_drain), io8_ft_i3c_spi_ls_1v8 (I/O_open_drain), io8_ft_i3c_spi_ls_3v3 (I/O_open_drain), io8_ft_i3c_spi_ms_1v2 (I/O_open_drain), io8_ft_i3c_spi_ms_1v8 (I/O_open_drain), io8_ft_i3c_spi_ms_3v3 (I/O_open_drain), io8_ft_i3c_spi_v33_fs_1v2 (I/O_open_drain), io8_ft_i3c_spi_v33_fs_1v8 (I/O_open_drain), io8_ft_i3c_spi_v33_fs_3v3 (I/O_open_drain), io8_ft_i3c_spi_v33_hs_1v2 (I/O_open_drain), io8_ft_i3c_spi_v33_hs_1v8 (I/O_open_drain), io8_ft_i3c_spi_v33_hs_3v3 (I/O_open_drain), io8_ft_i3c_spi_v33_ls_1v2 (I/O_open_drain), io8_ft_i3c_spi_v33_ls_1v8 (I/O_open_drain), io8_ft_i3c_spi_v33_ls_3v3 (I/O_open_drain), io8_ft_i3c_spi_v33_ms_1v2 (I/O_open_drain), io8_ft_i3c_spi_v33_ms_1v8 (I/O_open_drain), io8_ft_i3c_spi_v33_ms_3v3 (I/O_open_drain), io8_ft_spi_fs_1v2 (I/O), io8_ft_spi_fs_1v8 (I/O)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
